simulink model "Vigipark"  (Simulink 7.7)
settings: Solver=ode45  StartTime=0.0  StopTime=inf  MaxStep=0.05  RelTol=1e-3
PostLoadFcn:
  | Init;
undefined symbols (not defined in the file or in its folder): deg, kg, m, N, Partie_mobile, rad, RootGround, RootPart, s, socle, Vigipark
libraries: mblibv1 x10, simulink x3

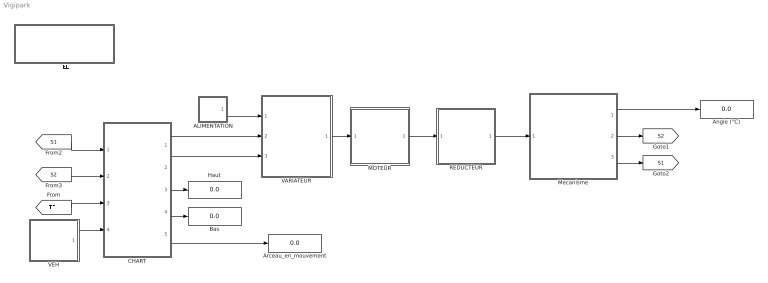
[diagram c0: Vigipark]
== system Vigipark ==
  ALIMENTATION : Subsystem  mask(PANNEAU PV - REGULATEUR DE CHARGE - BATTERIE){Ubat=12}
      mask prompts: Ubat "Tension batterie (V)"
      mask help: FONCTION : ALIMENTER
  Angle (°C) : Display
  Arceau_en_mouvement : Display
  Bas : Display
  CHART : Stateflow chart  TreatAsAtomicUnit=on
  Haut : Display
  MOTEUR : Subsystem  mask(MOTEUR ASYNCHRONE TRIPHASE){Nn=3700, Un=12}
      mask prompts: Nn "Vitesse nominale (tr/min)"; Un "Tension nominale (V)"
      mask help: Type de moteur
  Mecanisme : Subsystem
  REDUCTEUR : Subsystem  mask(REDUCTEUR A ENGRENAGES){Z1=20, Z2=44}
      mask prompts: Z1 "Nombre de dents Z1"; Z2 "Nombre de dents Z2"
      mask help: Nombre de dents des différentes roues
  TEL : Subsystem  mask{TEL=0}
      mask prompts: TEL "Télécommande sollicitée O/N"
  VARIATEUR : Subsystem
  VEH : Subsystem  mask{VEH=0}
      mask prompts: VEH "Vehicule présent / absent"
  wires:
  Mecanisme/1(Angle (°)) -> Angle (°C)/1
  [TEL] -> CHART/3(TEL)
  VEH/1(NL VEH) -> CHART/4(VEHICULE)
  Mecanisme/2(NL S2) -> [S2]
  Mecanisme/3(NL S1) -> [S1]
  [S1] -> CHART/1(S1)
  [S2] -> CHART/2(S2)
  REDUCTEUR/1(S) -> Mecanisme/1(N (tr/min))
  VARIATEUR/1(OUT) -> MOTEUR/1(IN)
  CHART/2(VIT) -> VARIATEUR/3(VITESSE)
  CHART/1(SENS) -> VARIATEUR/2(SENS)
  ALIMENTATION/1(OUT) -> VARIATEUR/1(ALIM)
  MOTEUR/1(OUT) -> REDUCTEUR/1(E)
  CHART/3(Haut) -> Haut/1
  CHART/4(Bas) -> Bas/1
  CHART/5(Move) -> Arceau_en_mouvement/1

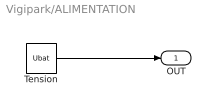
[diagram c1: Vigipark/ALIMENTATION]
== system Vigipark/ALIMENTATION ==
  Tension : Constant  Value=Ubat
  OUT : Outport
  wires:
  Tension/1 -> OUT/1

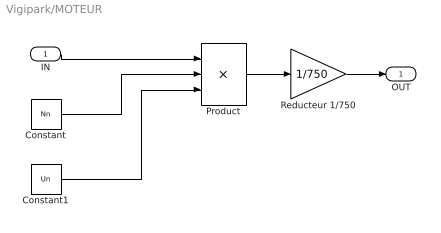
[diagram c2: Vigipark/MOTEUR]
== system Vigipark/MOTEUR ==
  IN : Inport
  Constant : Constant  Value=Nn
  Constant1 : Constant  Value=Un
  Product : Product  Inputs=**/
  Reducteur 1/750 : Gain  Gain=1/750
  OUT : Outport
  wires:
  IN/1 -> Product/1
  Constant/1 -> Product/2
  Constant1/1 -> Product/3
  Product/1 -> Reducteur 1/750/1
  Reducteur 1/750/1 -> OUT/1

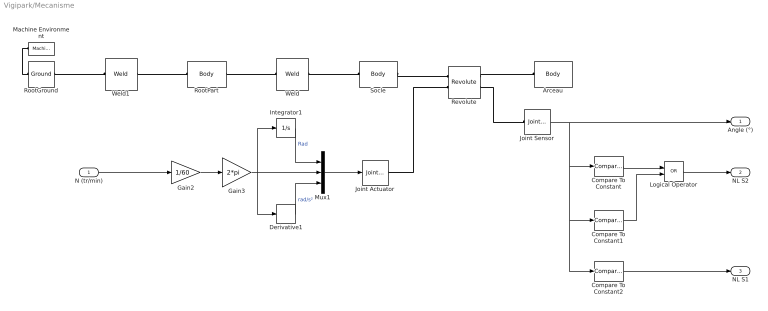
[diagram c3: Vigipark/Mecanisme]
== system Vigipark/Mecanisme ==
  N (tr/min) : Inport
  Arceau : mblibv1/Bodies/Body  PhysicalDomain=mechanical  SubClassName=Unknown  LeftPortType=workingframe  RightPortType=workingframe  LConnTagsString=CS2  UpdateFromCAD=on  PMImportedID=Partie_mobile-1  DialogClass=MechanicalBodyBlock  Mass=32.744  MassUnits=kg  InertiaUnits=kg*m^2  Inertia=[1.00541,-3.3552e-005,2.30229e-006;-3.3552e-005,1.97826,-0.0120003;2.30229e-006,-0.0120003,2.9678]  Shape=Cylinder  ShapeDims=[1 1]  ShapeUnits=m  ShapeUse=false  Density=1  DensityUnits=kg/m^3  DensityUse=false  GraphicsMode=GFXFILE  GraphicsFileName=Arceau.STL  BodyColorSelMode=COLORPALETTE  BodyColor=[0.75294 0.75294 0.75294]  AttachedToCS=CS1  CG=Right$CG$[-0.0264843 0.450269 -0.149943]$WORLD$WORLD$m$[1 0 0;0 0.999928 0.0119791;0 -0.0119791 0.999928]$3x3 Transform$rad$WORLD$false$Partie_mobile-1::CG(AUTOGEN)  WorkingFrames=Right$CS1$[-0.248449 0.0248812 0.39294]$WORLD$WORLD$m$[1 0 0;0 0.999928 0.0119791;0 -0.0119791 0.999928]$3x3 Transform$rad$WORLD$false$Partie_mobile-1::CS1(AUTOGEN)#Left$CS2$[0.191141 0.0583797 -0.15]$WORLD$WORLD$m$[1 0 0;0 1 0;0 0 1]$3x3 Transform$rad$WORLD$true$Partie_mobile-1:-:socle-1::Partie_mobile-1(AUTOGEN)  CGPos=[-0.0264843 0.450269 -0.149943]  CGRot=[1 0 0;0 0.999928 0.0119791;0 -0.0119791 0.999928]  CS0Pos=[]  CS0Rot=[]  CS1Pos=[-0.248449 0.0248812 0.39294]  CS1Rot=[1 0 0;0 0.999928 0.0119791;0 -0.0119791 0.999928]  CS2Pos=[0.191141 0.0583797 -0.15]  CS2Rot=[1 0 0;0 1 0;0 0 1]  CS3Pos=[]  CS3Rot=[]  CS4Pos=[]  CS4Rot=[]  CS5Pos=[]  CS5Rot=[]  CS6Pos=[]  CS6Rot=[]  CS7Pos=[]  CS7Rot=[]  CS8Pos=[]  CS8Rot=[]  CS9Pos=[]  CS9Rot=[]  CS10Pos=[]  CS10Rot=[]  CS11Pos=[]  CS11Rot=[]  CS12Pos=[]  CS12Rot=[]  CS13Pos=[]  CS13Rot=[]  CS14Pos=[]  CS14Rot=[]  CS15Pos=[]  CS15Rot=[]  CS16Pos=[]  CS16Rot=[]  CS17Pos=[]  CS17Rot=[]  CS18Pos=[]  CS18Rot=[]  CS19Pos=[]  CS19Rot=[]  CS20Pos=[]  CS20Rot=[]
  Compare To Constant : simulink/Logic and Bit Operations/Compare To Constant  SystemSampleTime=-1  relop=<=  const=2  LogicOutDataTypeMode=boolean
  Compare To Constant1 : simulink/Logic and Bit Operations/Compare To Constant  SystemSampleTime=-1  relop=>=  const=88  LogicOutDataTypeMode=boolean
  Compare To Constant2 : simulink/Logic and Bit Operations/Compare To Constant  SystemSampleTime=-1  relop=>=  const=44  LogicOutDataTypeMode=boolean
  Derivative1 : Derivative
  Gain2 : Gain  Gain=1/60
  Gain3 : Gain  Gain=2*pi
  Integrator1 : Integrator
  Joint Actuator : mblibv1/Sensors &  Actuators/Joint Actuator  SystemSampleTime=-1  UpdateFromCAD=off  PhysicalDomain=Mechanical  PortType=blob  ActuationStyle=Motion  AngleUnits=rad  ArcVelocityUnits=rad/s  ArcAccelerationUnits=rad/s^2  CoordPositionUnits=m  VelocityUnits=m/s  AccelerationUnits=m/s^2  ForceUnits=N  TorqueUnits=N*m  ActiveIO=on  Width=3  DialogClass=MechanicalActuatorBlock  Primitive=R1  ReferenceFrame=Absolute (World)
  Joint Sensor : mblibv1/Sensors &  Actuators/Joint Sensor  SystemSampleTime=-1  UpdateFromCAD=off  PhysicalDomain=Mechanical  PortType=blob  Muxed=on  Pose=off  Angle=on  AngleUnits=deg  ArcVelocity=off  ArcVelocityUnits=deg/s  ArcAcceleration=off  ArcAccelerationUnits=deg/s^2  CoordPosition=on  CoordPositionUnits=m  Velocity=off  VelocityUnits=m/s  Acceleration=off  AccelerationUnits=m/s^2  Quaternion=on  QuaternionDT=off  QuaternionDDT=off  QuaternionUnits=off  OutputVector=[1]  ActiveIO=on  Width=1  DialogClass=MechanicalSensorBlock  Primitive=R1  Force=off  ForceUnits=N  Torque=off  TorqueUnits=N*m  ReferenceFrame=Absolute (World)  ReactionSensedSide=Base  ReactionReferenceFrame=Absolute (World)  ReactionForce=off  ReactionForceUnits=N  ReactionMoment=off  ReactionMomentUnits=N*m
  Logical Operator : Logic  Operator=OR  AllPortsSameDT=off  OutDataTypeStr=boolean
  Machine Environment : mblibv1/Bodies/Machine Environment  SystemSampleTime=-1  PortType=env  PhysicalDomain=Mechanical  DialogTemplateClass=MECH.MachineEnvironment  SyncWhenCopied=off  Gravity=[0 -9.81 0]  GravityUnits=m/s^2  GravityAsSignal=off  Dimensionality=Auto-detect  AnalysisType=Forward dynamics  LinearAssemblyTolerance=1e-3  LinearAssemblyToleranceUnits=m  AngularAssemblyTolerance=1e-3  AngularAssemblyToleranceUnits=rad  ConstraintSolverType=Stabilizing  ConstraintRelTolerance=1e-4  ConstraintAbsTolerance=1e-4  UseRobustSingularityHandling=off  RedundancyAnalysisToleranceType=Automatically select tolerance  RedundancyAnalysisTolerance=1e-14  StatePerturbationType=Fixed  PerturbationSize=1e-5  VisualizeMachine=on  BodyVisualizationType=Use model default body geometries  BodyColorSelMode=Use model default  DefaultBodyColor=[1 0 0]
  Mux1 : Mux  Inputs=3
  Revolute : mblibv1/Joints/Revolute  PhysicalDomain=mechanical  SubClassName=Unknown  LeftPortType=blob  RightPortType=blob  LConnTagsString=__newl0|SA1  RConnTagsString=__newr0|SA1  UpdateFromCAD=on  PMImportedID=Partie_mobile-1:-:socle-1  NumSAPorts=2  CutJoint=off  MarkAsCut=off  Primitives=prismatic  PrimitiveProps=R1$World$[1,0,0]$revolute  DialogClass=JointBlock  R1Axis=[1,0,0]
  RootGround : mblibv1/Bodies/Ground  SystemSampleTime=-1  UpdateFromCAD=on  PMImportedID=RootGround  LeftPortType=env  RightPortType=workingframe  PhysicalDomain=Mechanical  DialogClass=GroundBlock  CoordPosition=[-0.0265495,0.439421,-0.145405]  CoordPositionUnits=m  StateVectorMgrId=0  MachineId=[1 0]  ShowEnvPort=on
  RootPart : mblibv1/Bodies/Body  PhysicalDomain=mechanical  SubClassName=Unknown  LeftPortType=workingframe  RightPortType=workingframe  LConnTagsString=CS3  RConnTagsString=CS2  UpdateFromCAD=on  PMImportedID=Vigipark/RootPart  DialogClass=MechanicalBodyBlock  Mass=0  MassUnits=kg  InertiaUnits=kg*m^2  Inertia=[0,0,0;0,0,0;0,0,0]  Shape=Cylinder  ShapeDims=[1 1]  ShapeUnits=m  ShapeUse=false  Density=1  DensityUnits=kg/m^3  DensityUse=false  GraphicsMode=MACHINE_DEFAULT  BodyColorSelMode=MACHINE_DEFAULT  BodyColor=[1;0;0]  AttachedToCS=CS1  CG=Right$CG$[-0.0265495 0.439421 -0.145405]$WORLD$WORLD$m$[1 0 0;0 1 0;0 0 1]$3x3 Transform$rad$WORLD$false$Vigipark/RootPart::CG(AUTOGEN)  WorkingFrames=Right$CS1$[0 0 0]$WORLD$WORLD$m$[1 0 0;0 1 0;0 0 1]$3x3 Transform$rad$WORLD$false$Vigipark/RootPart::CS1(AUTOGEN)#Right$CS2$[-0.0287729 0.0693234 0.00940228]$WORLD$WORLD$m$[1 0 0;0 1 0;0 0 1]$3x3 Transform$rad$WORLD$true$Vigipark/RootPart:-:socle-1::Vigipark/RootPart(AUTOGEN)#Left$CS3$[-0.0265495 0.439421 -0.145405]$WORLD$WORLD$m$[1 0 0;0 1 0;0 0 1]$3x3 Transform$rad$WORLD$true$RootGround:-:Vigipa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  CGPos=[-0.0265495 0.439421 -0.145405]  CGRot=[1 0 0;0 1 0;0 0 1]  CS0Pos=[]  CS0Rot=[]  CS1Pos=[0 0 0]  CS1Rot=[1 0 0;0 1 0;0 0 1]  CS2Pos=[-0.0287729 0.0693234 0.00940228]  CS2Rot=[1 0 0;0 1 0;0 0 1]  CS3Pos=[-0.0265495 0.439421 -0.145405]  CS3Rot=[1 0 0;0 1 0;0 0 1]  CS4Pos=[]  CS4Rot=[]  CS5Pos=[]  CS5Rot=[]  CS6Pos=[]  CS6Rot=[]  CS7Pos=[]  CS7Rot=[]  CS8Pos=[]  CS8Rot=[]  CS9Pos=[]  CS9Rot=[]  CS10Pos=[]  CS10Rot=[]  CS11Pos=[]  CS11Rot=[]  CS12Pos=[]  CS12Rot=[]  CS13Pos=[]  CS13Rot=[]  CS14Pos=[]  CS14Rot=[]  CS15Pos=[]  CS15Rot=[]  CS16Pos=[]  CS16Rot=[]  CS17Pos=[]  CS17Rot=[]  CS18Pos=[]  CS18Rot=[]  CS19Pos=[]  CS19Rot=[]  CS20Pos=[]  CS20Rot=[]
  Socle : mblibv1/Bodies/Body  PhysicalDomain=mechanical  SubClassName=Unknown  LeftPortType=workingframe  RightPortType=workingframe  LConnTagsString=CS2  RConnTagsString=CS3  UpdateFromCAD=on  PMImportedID=socle-1  DialogClass=MechanicalBodyBlock  Mass=0.95983  MassUnits=kg  InertiaUnits=kg*m^2  Inertia=[0.0419737,-1.37018e-005,9.40934e-005;-1.37018e-005,0.0619611,0.000613274;9.40934e-005,0.000613274,0.021331]  Shape=Cylinder  ShapeDims=[1 1]  ShapeUnits=m  ShapeUse=false  Density=1  DensityUnits=kg/m^3  DensityUse=false  GraphicsMode=GFXFILE  GraphicsFileName=Socle.STL  BodyColorSelMode=COLORPALETTE  BodyColor=[0.50196 0.50196 1]  AttachedToCS=CS1  CG=Right$CG$[-0.0287729 0.0693234 0.00940228]$WORLD$WORLD$m$[1 0 0;0 1 0;0 0 1]$3x3 Transform$rad$WORLD$false$socle-1::CG(AUTOGEN)  WorkingFrames=Right$CS1$[-0.027859 0.0183797 0.375]$WORLD$WORLD$m$[1 0 0;0 1 0;0 0 1]$3x3 Transform$rad$WORLD$false$socle-1::CS1(AUTOGEN)#Left$CS2$[-0.0287729 0.0693234 0.00940228]$WORLD$WORLD$m$[1 0 0;0 1 0;0 0 1]$3x3 Transform$rad$WORLD$true$Vigipark/RootPart:-:socle-1::socle-1(AUTOGEN)#Right$CS3$[0.191141 0.0583797 -0.15]$WORLD$WORLD$m$[1 0 0;0 1 0;0 0 1]$3x3 Transform$rad$WORLD$true$Partie_mobile-1:-:socle-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  CGPos=[-0.0287729 0.0693234 0.00940228]  CGRot=[1 0 0;0 1 0;0 0 1]  CS0Pos=[]  CS0Rot=[]  CS1Pos=[-0.027859 0.0183797 0.375]  CS1Rot=[1 0 0;0 1 0;0 0 1]  CS2Pos=[-0.0287729 0.0693234 0.00940228]  CS2Rot=[1 0 0;0 1 0;0 0 1]  CS3Pos=[0.191141 0.0583797 -0.15]  CS3Rot=[1 0 0;0 1 0;0 0 1]  CS4Pos=[]  CS4Rot=[]  CS5Pos=[]  CS5Rot=[]  CS6Pos=[]  CS6Rot=[]  CS7Pos=[]  CS7Rot=[]  CS8Pos=[]  CS8Rot=[]  CS9Pos=[]  CS9Rot=[]  CS10Pos=[]  CS10Rot=[]  CS11Pos=[]  CS11Rot=[]  CS12Pos=[]  CS12Rot=[]  CS13Pos=[]  CS13Rot=[]  CS14Pos=[]  CS14Rot=[]  CS15Pos=[]  CS15Rot=[]  CS16Pos=[]  CS16Rot=[]  CS17Pos=[]  CS17Rot=[]  CS18Pos=[]  CS18Rot=[]  CS19Pos=[]  CS19Rot=[]  CS20Pos=[]  CS20Rot=[]
  Weld : mblibv1/Joints/Weld  PhysicalDomain=mechanical  SubClassName=Unknown  LeftPortType=blob  RightPortType=blob  LConnTagsString=__newl0  RConnTagsString=__newr0  UpdateFromCAD=on  PMImportedID=Vigipark/RootPart:-:socle-1  NumSAPorts=0  CutJoint=off  MarkAsCut=off  Primitives=weld  PrimitiveProps=W$WORLD$[0.57735,0.57735,0.57735]$weld  DialogClass=JointBlock  WAxis=[0.57735,0.57735,0.57735]
  Weld1 : mblibv1/Joints/Weld  PhysicalDomain=mechanical  SubClassName=Unknown  LeftPortType=blob  RightPortType=blob  LConnTagsString=__newl0  RConnTagsString=__newr0  UpdateFromCAD=on  PMImportedID=RootGround:-:Vigipark/RootPart  NumSAPorts=0  CutJoint=off  MarkAsCut=off  Primitives=weld  PrimitiveProps=W$WORLD$[0.57735,0.57735,0.57735]$weld  DialogClass=JointBlock  WAxis=[0.57735,0.57735,0.57735]
  Angle (°) : Outport
  NL S2 : Outport  Port=2
  NL S1 : Outport  Port=3
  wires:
  Integrator1/1 -> Mux1/1  "Rad"
  Derivative1/1 -> Mux1/3  "rad/s²"
  Gain3/1 -> Mux1/2, Derivative1/1, Integrator1/1
  Mux1/1 -> Joint Actuator/1
  Gain2/1 -> Gain3/1
  N (tr/min)/1 -> Gain2/1
  Joint Sensor/1 -> Angle (°)/1, Compare To Constant/1, Compare To Constant1/1, Compare To Constant2/1
  Compare To Constant/1 -> Logical Operator/1
  Logical Operator/1 -> NL S2/1
  Compare To Constant1/1 -> Logical Operator/2
  Compare To Constant2/1 -> NL S1/1
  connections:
  Revolute/RConn1 -- Arceau/LConn1
  Joint Actuator/RConn1 -- Revolute/LConn2
  Revolute/RConn2 -- Joint Sensor/LConn1
  RootGround/LConn1 -- Machine Environment/RConn1
  Socle/RConn1 -- Revolute/LConn1
  RootGround/RConn1 -- Weld1/LConn1
  Weld1/RConn1 -- RootPart/LConn1
  RootPart/RConn1 -- Weld/LConn1
  Weld/RConn1 -- Socle/LConn1

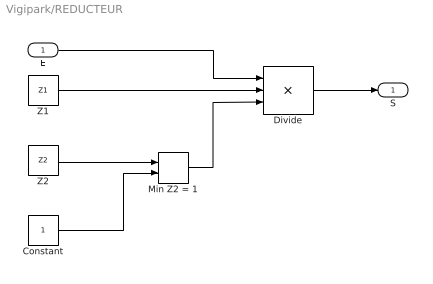
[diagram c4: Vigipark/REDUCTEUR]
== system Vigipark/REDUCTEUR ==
  E : Inport
  Constant : Constant
  Divide : Product  Inputs=**/
  Min Z2 = 1 : MinMax  Function=max  Inputs=2
  Z1 : Constant  Value=Z1
  Z2 : Constant  Value=Z2
  S : Outport
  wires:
  Z1/1 -> Divide/2
  Divide/1 -> S/1
  Constant/1 -> Min Z2 = 1/2
  Z2/1 -> Min Z2 = 1/1
  Min Z2 = 1/1 -> Divide/3
  E/1 -> Divide/1

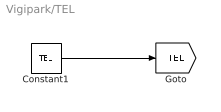
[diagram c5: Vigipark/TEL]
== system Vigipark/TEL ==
  Constant1 : Constant  Value=TEL
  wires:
  Constant1/1 -> [TEL]

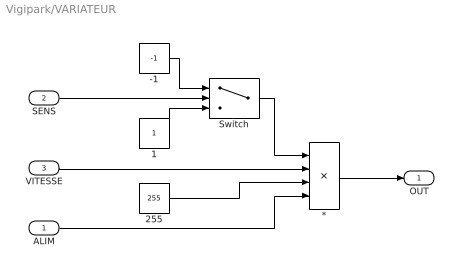
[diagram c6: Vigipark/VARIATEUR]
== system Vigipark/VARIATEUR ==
  ALIM : Inport
  SENS : Inport  Port=2
  VITESSE : Inport  Port=3
  * : Product  Inputs=**/*
  -1 : Constant  Value=-1
  1 : Constant
  255 : Constant  Value=255
  Switch : Switch  Threshold=0.5
  OUT : Outport
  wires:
  VITESSE/1 -> */2
  SENS/1 -> Switch/2
  Switch/1 -> */1
  -1/1 -> Switch/1
  1/1 -> Switch/3
  */1 -> OUT/1
  255/1 -> */3
  ALIM/1 -> */4

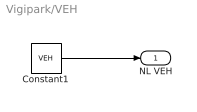
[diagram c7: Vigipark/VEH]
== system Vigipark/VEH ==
  Constant1 : Constant  Value=VEH
  NL VEH : Outport
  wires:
  Constant1/1 -> NL VEH/1

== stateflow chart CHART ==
  state EN_SERVICE
    state COMMANDE
      state ARRET
        entry: VIT=0;
      state DESC_debut
        entry:
      state DESC_fin
      state MONT_debut
        entry:
      state MONT_fin
      (default) -> ARRET
      ARRET -> MONT_debut
      DESC_fin -> ARRET
      MONT_fin -> ARRET : [S2]
      ARRET -> DESC_debut : [TEL & !S1]
      DESC_debut -> DESC_fin
      MONT_debut -> MONT_fin
    (default) -> COMMANDE
  (default) -> EN_SERVICE
